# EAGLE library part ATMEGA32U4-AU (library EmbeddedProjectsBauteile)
ATMEL 8-bit Microcontroller with 16/32K Bytes of ISP Flash and USB Controller
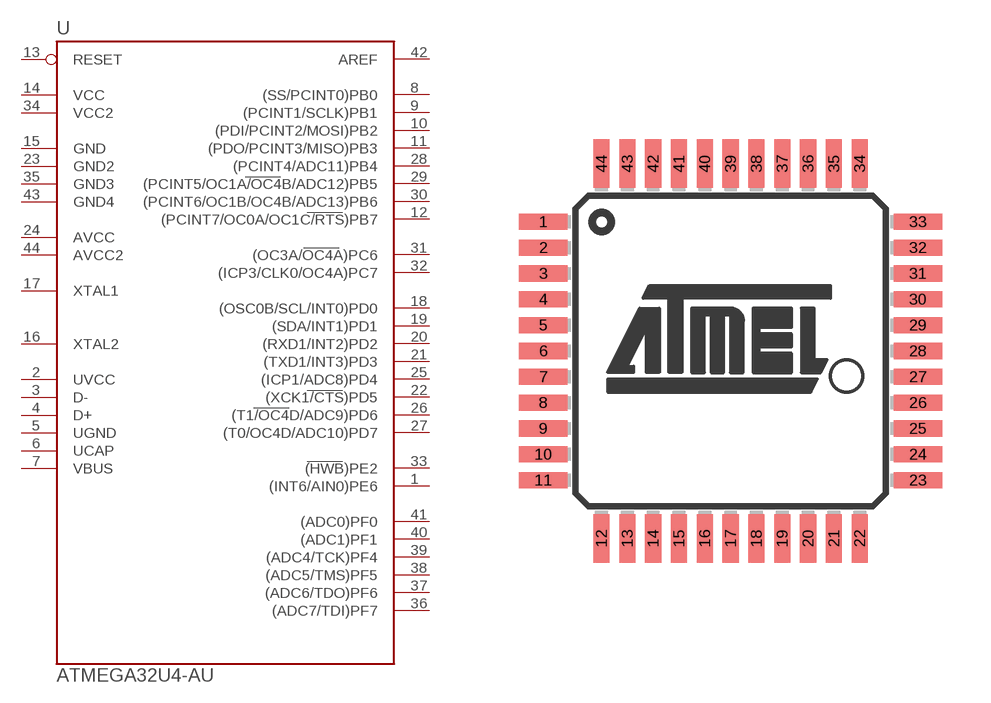
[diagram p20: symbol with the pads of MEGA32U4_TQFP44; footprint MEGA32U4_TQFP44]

Designator prefix -

## ATMEGA32U4-AU (EP: 400297)  [MEGA32U4_TQFP44]
1  (INT6/AIN0)PE6
2  UVCC
3  D-
4  D+
5  UGND
6  UCAP
7  VBUS
8  (SS/PCINT0)PB0
9  (PCINT1/SCLK)PB1
10  (PDI/PCINT2/MOSI)PB2
11  (PDO/PCINT3/MISO)PB3
12  (PCINT7/OC0A/OC1C/RTS)PB7
13  RESET
14  VCC
15  GND
16  XTAL2
17  XTAL1
18  (OSC0B/SCL/INT0)PD0
19  (SDA/INT1)PD1
20  (RXD1/INT2)PD2
21  (TXD1/INT3)PD3
22  (XCK1/CTS)PD5
23  GND2
24  AVCC
25  (ICP1/ADC8)PD4
26  (T1/OC4D/ADC9)PD6
27  (T0/OC4D/ADC10)PD7
28  (PCINT4/ADC11)PB4
29  (PCINT5/OC1A/OC4B/ADC12)PB5
30  (PCINT6/OC1B/OC4B/ADC13)PB6
31  (OC3A/OC4A)PC6
32  (ICP3/CLK0/OC4A)PC7
33  (HWB)PE2
34  VCC2
35  GND3
36  (ADC7/TDI)PF7
37  (ADC6/TDO)PF6
38  (ADC5/TMS)PF5
39  (ADC4/TCK)PF4
40  (ADC1)PF1
41  (ADC0)PF0
42  AREF
43  GND4
44  AVCC2

## Footprint MEGA32U4_TQFP44 (pad centres in mm)
Thin Plasic Quad Flat Package
smd 1.5 x 0.5: 1 -5.8,4; 2 -5.8,3.2; 3 -5.8,2.4; 4 -5.8,1.6; 5 -5.8,0.8; 6 -5.8,0; 7 -5.8,-0.8; 8 -5.8,-1.6; 9 -5.8,-2.4; 10 -5.8,-3.2; 11 -5.8,-4; 23 5.8,-4; 24 5.8,-3.2; 25 5.8,-2.4; 26 5.8,-1.6; 27 5.8,-0.8; 28 5.8,0; 29 5.8,0.8; 30 5.8,1.6; 31 5.8,2.4; 32 5.8,3.2; 33 5.8,4
smd 0.5 x 1.5: 12 -4,-5.8; 13 -3.2,-5.8; 14 -2.4,-5.8; 15 -1.6,-5.8; 16 -0.8,-5.8; 17 0,-5.8; 18 0.8,-5.8; 19 1.6,-5.8; 20 2.4,-5.8; 21 3.2,-5.8; 22 4,-5.8; 34 4,5.8; 35 3.2,5.8; 36 2.4,5.8; 37 1.6,5.8; 38 0.8,5.8; 39 0,5.8; 40 -0.8,5.8; 41 -1.6,5.8; 42 -2.4,5.8; 43 -3.2,5.8; 44 -4,5.8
